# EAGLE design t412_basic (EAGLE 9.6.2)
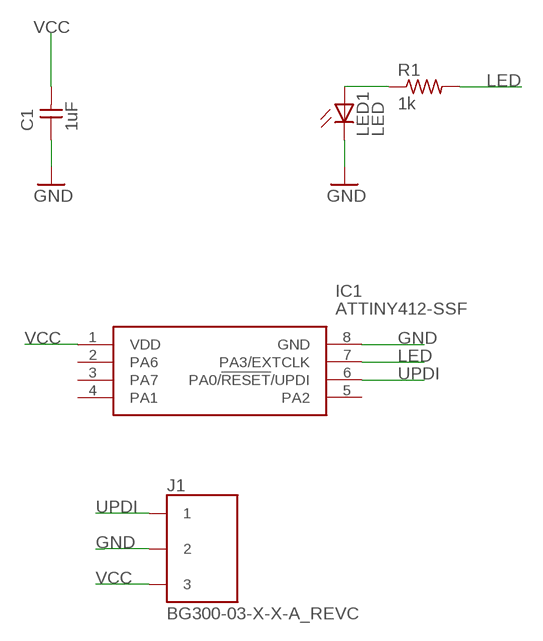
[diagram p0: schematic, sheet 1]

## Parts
C1  1uF  CAP_UNPOLARIZED  [C1206]
IC1  ATTINY412-SSF  [SOIC127P600X175-8N]
J1  BG300-03-X-X-A_REVC  [GCT_BG300-03-X-X-A_REVC]
LED1  LED  [LED1206]
R1  1k  R1206  [R1206]

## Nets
GND: C1.1 IC1.8(GND) J1.2 LED1.2(C)
LED: IC1.7(PA3/EXTCLK) R1.2
N$13: LED1.1(A) R1.1
UPDI: IC1.6(PA0/!RESET!/UPDI) J1.1
VCC: C1.2 IC1.1(VDD) J1.3
Unconnected: IC1.2(PA6) IC1.3(PA7) IC1.4(PA1) IC1.5(PA2)

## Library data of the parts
C1 = fab:CAP_UNPOLARIZED
IC1 = ATTINY412-SSF:ATTINY412-SSF: 8-bit Microcontrollers - MCU 20MHz, 4KB, SOIC8, Ind 125C, Green, Tube Source: Datasheet; DESCRIPTION: 8-bit Microcontrollers - MCU 20MHz, 4KB, SOIC8, Ind 125C, Green, Tube; HEIGHT: 1.75mm; MANUFACTURER_NAME: Microchip; MANUFACTURER_PART_NUMBER: ATTINY412-SSF; MOUSER_PART_NUMBER: 579-ATTINY412-SSF; MOUSER_PRICE-STOCK: https://www.mouser.com/Search/Refine.aspx?Keyword=579-ATTINY412-SSF
J1 = BG300-03-X-X-A_REVC:BG300-03-X-X-A_REVC: 2.54mm Pitch Socket, Single Row, Surface Mount, Horizontal, Natural LCP; MANUFACTURER: GCT
LED1 = fab:LED: LED
R1 = fab:R: Resistor (US Symbol)

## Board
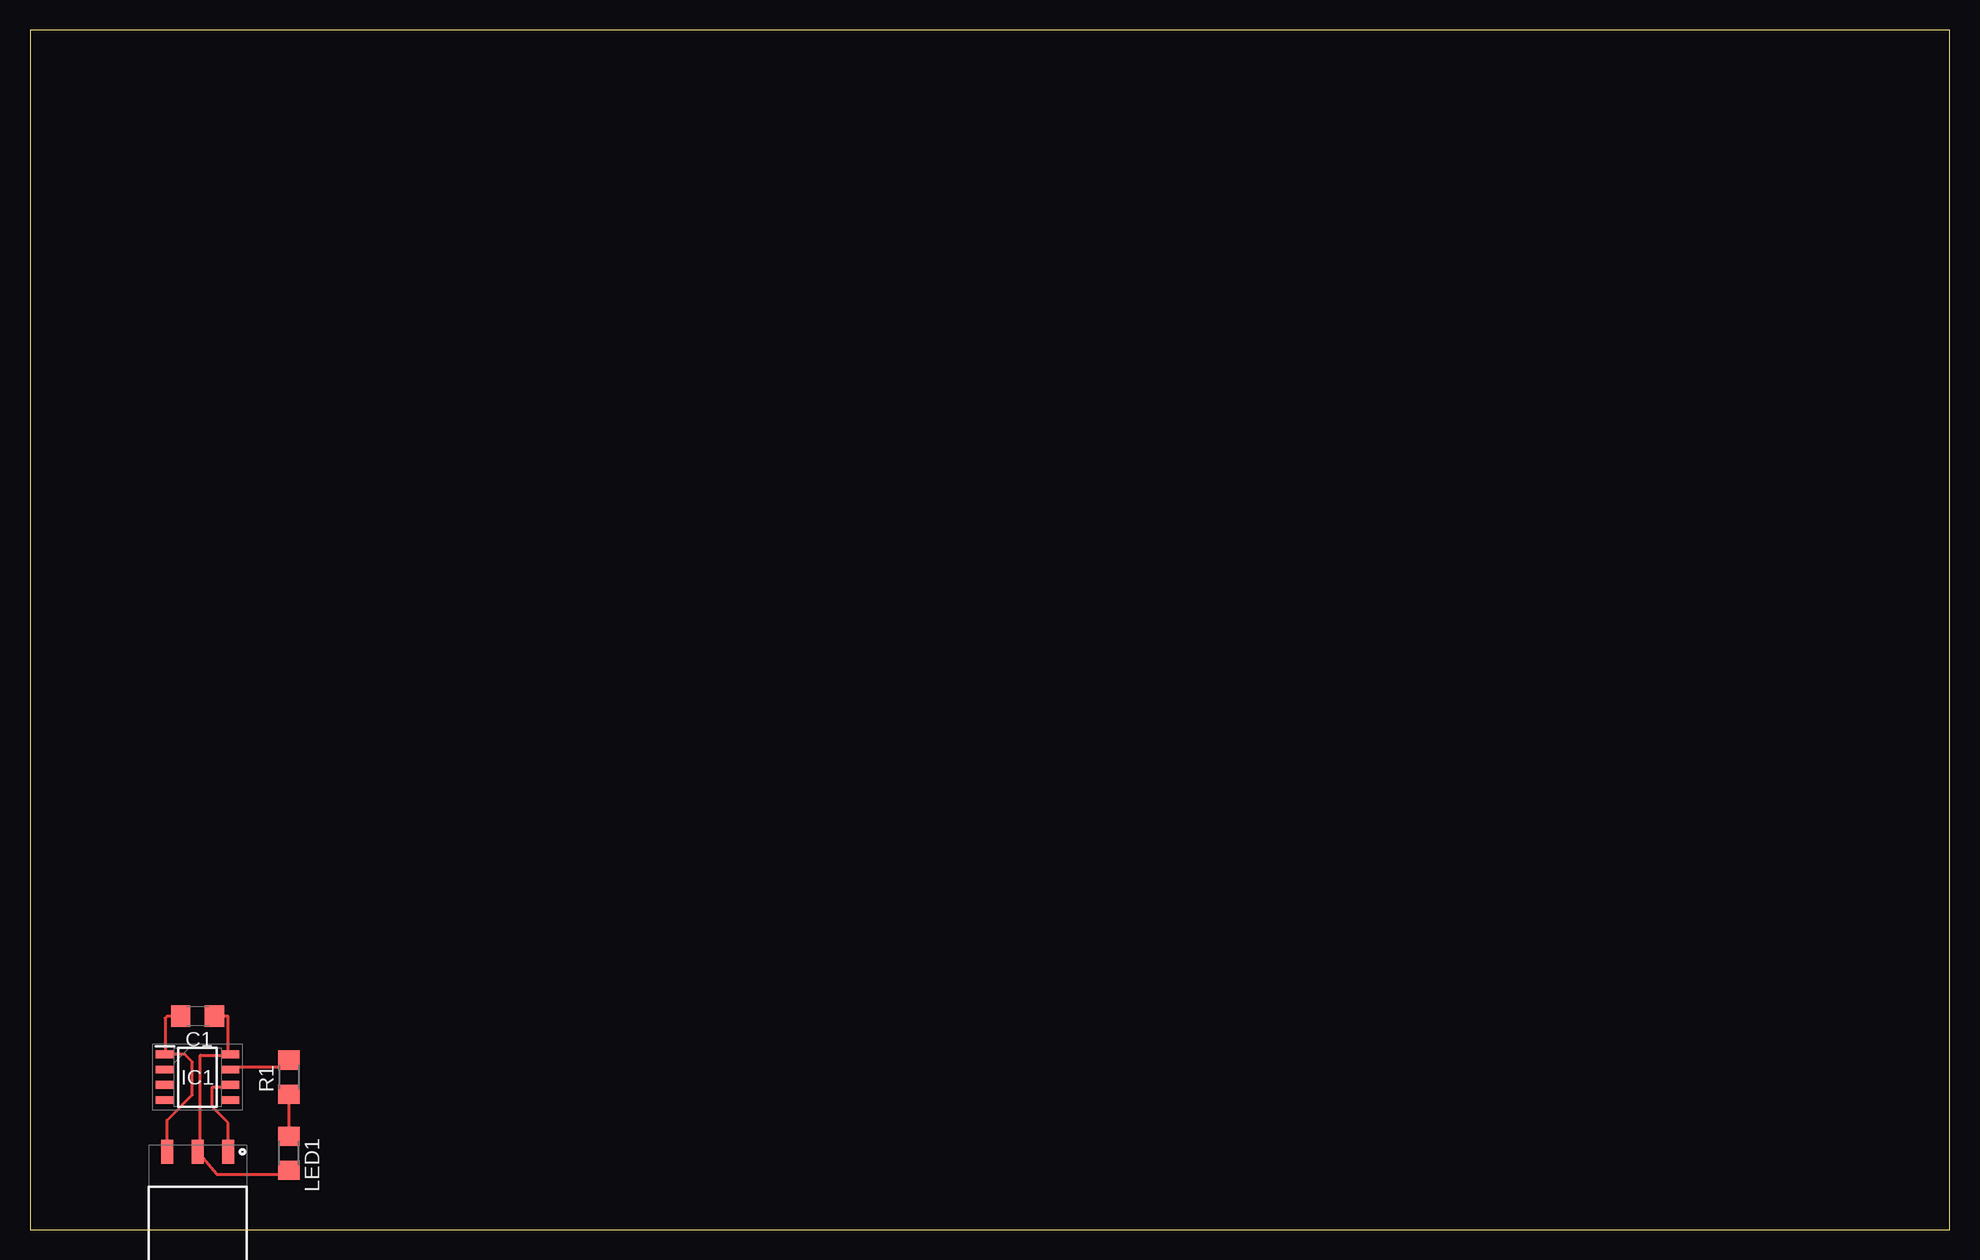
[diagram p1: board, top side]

Size 160 x 100 mm. Coordinates in mm from the lower left corner, seen from the top.
Outline: 0,0 160,0 160,100 0,100 0,0
Copper layers (1*16): Top 0.035mm / dielectric 1.5mm / Bottom 0.035mm
Design rules "fab": minimum track width 10mil, minimum drill 32mil, track to track 16mil, track to pad 16mil, pad to pad 16mil, via to via 16mil, smd to smd 6mil, copper to edge 16mil, drill to drill 16mil, minimum pad ring 10mil, minimum via ring 8mil, stop-mask expansion 4mil, vias tented up to drill 0mil, thermal gap 16mil

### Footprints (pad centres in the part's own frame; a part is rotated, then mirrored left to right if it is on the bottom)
C1206 = smd 1.6 x 1.8: 1 -1.4,0; 2 1.4,0
SOIC127P600X175-8N = smd 1.525 x 0.65: 1 -2.712,1.905; 2 -2.712,0.635; 3 -2.712,-0.635; 4 -2.712,-1.905; 5 2.712,-1.905; 6 2.712,-0.635; 7 2.712,0.635; 8 2.712,1.905
GCT_BG300-03-X-X-A_REVC = smd 1 x 2: 1 -2.54,-5.225; 2 0,-5.225; 3 2.54,-5.225
LED1206 = smd 1.6 x 1.803: 1 -1.422,0; 2 1.422,0
R1206 = smd 1.6 x 1.803: 1 -1.422,0; 2 1.422,0

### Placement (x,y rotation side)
C1  13.97,17.78 180 top
IC1  13.97,12.7 0 top
J1  13.97,1.27 180 top
LED1  21.59,6.35 270 top
R1  21.59,12.7 90 top

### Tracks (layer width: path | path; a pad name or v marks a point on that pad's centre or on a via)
GND
  Top 0.254: 16.51,14.86 IC1.8 | 15.52,17.5 C1.1 16.51,17.78 16.51,14.78 IC1.8 | LED1.2 21.46,4.62 15.54,4.62 J1.2 14.2,6.55 14.2,14.53 16.51,14.53 IC1.8
LED
  Top 0.254: IC1.7 16.84,13.54 21.13,13.54 21.46,13.87 R1.2
N$13
  Top 0.254: 21.79,11.23 R1.1 LED1.1
UPDI
  Top 0.254: IC1.6 16.51,11.89 15.19,11.89 15.19,10.21 16.51,8.89 J1.1
VCC
  Top 0.254: 11.56,6.55 J1.3 11.43,9.12 13.54,11.23 13.54,13.97 12.9,14.61 IC1.1 11.26,17.61 11.43,17.78 C1.2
